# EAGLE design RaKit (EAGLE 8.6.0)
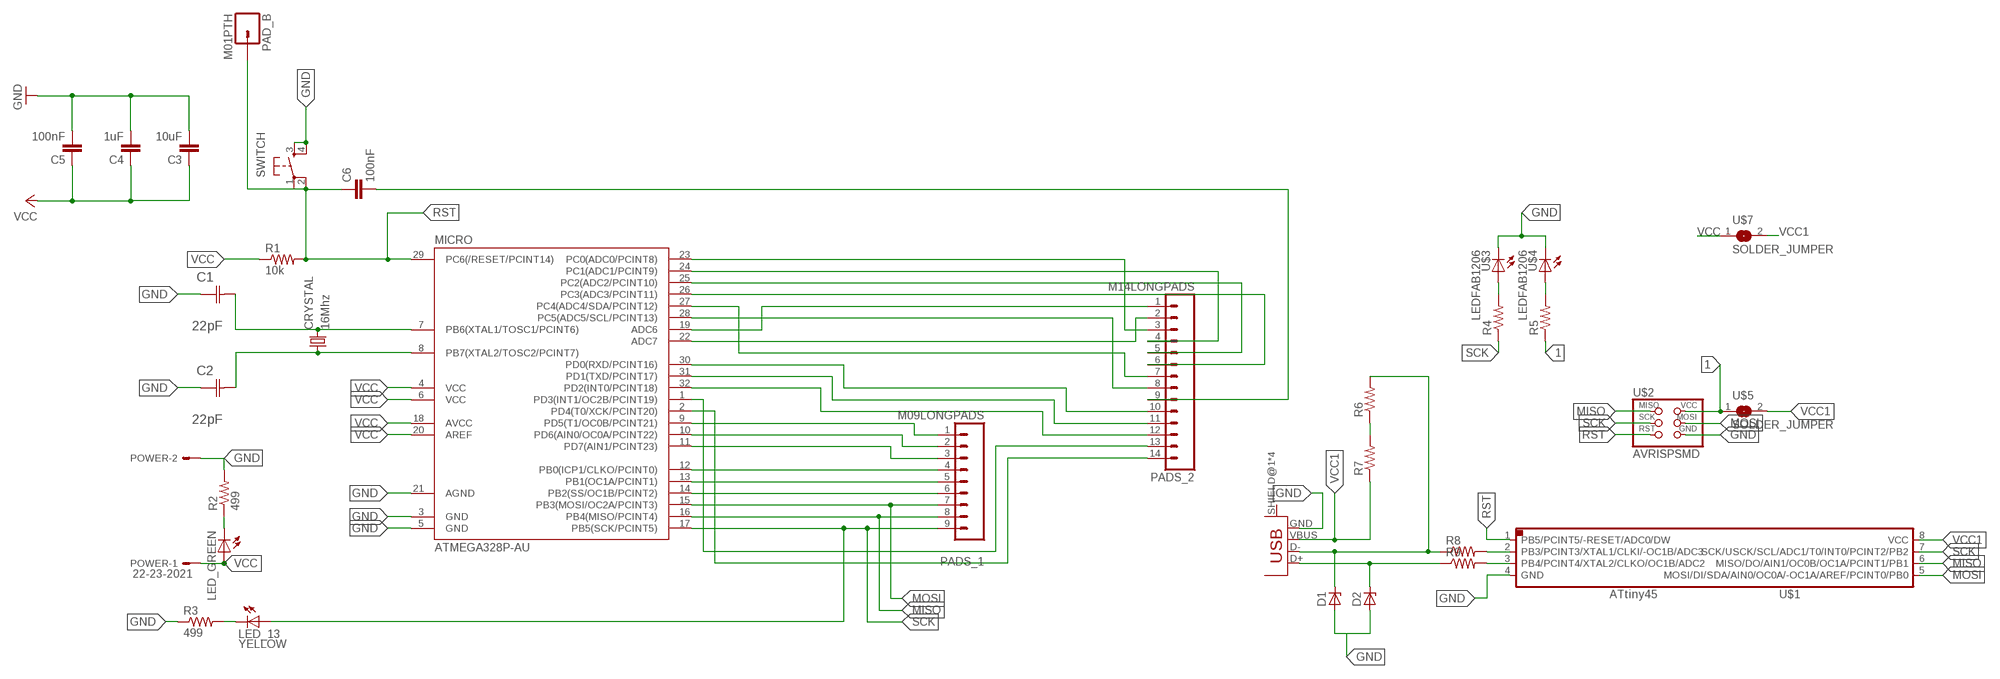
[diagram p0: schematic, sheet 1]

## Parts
C1  22pF  0612ZC225MAT2A  [CAPC3216X178N]
C2  22pF  0612ZC225MAT2A  [CAPC3216X178N]
C3  10uF  CAP1206  [1206]
C4  1uF  CAP1206  [1206]
C5  100nF  CAP1206  [1206]
C6  100nF  CAP1206  [1206]
CRYSTAL  16Mhz  CSM-7X-DU  [CSM-7X-DU]
D1  ZENER_DIODESOD123  [SOD123]
D2  ZENER_DIODESOD123  [SOD123]
LED_13  YELLOW  LED1206  [1206]
LED_GREEN  LED1206  [1206]
MICRO  ATMEGA328P-AU  ATMEGA48/88/168-AU  [TQFP32-08]
PAD_B  M01PTH  [1X01]
PADS_1  M09LONGPADS  [1X09_LONGPADS]
PADS_2  M14LONGPADS  [1X14-LONGPADS]
POWER  22-23-2021  [22-23-2021]
R1  10k  RESISTOR1206  [1206]
R2  499  RESISTOR1206  [1206]
R3  499  RESISTOR1206  [1206]
R4  RES-US1206FAB  [R1206FAB]
R5  RES-US1206FAB  [R1206FAB]
R6  RES-US1206FAB  [R1206FAB]
R7  RES-US1206FAB  [R1206FAB]
R8  RES-US1206FAB  [R1206FAB]
R9  RES-US1206FAB  [R1206FAB]
SWITCH  6MM_SWITCH6MM_SWITCH  [6MM_SWITCH]
U$1  ATTINY45SI  [SOIC8]
U$2  AVRISPSMD  [2X03SMD]
U$3  LEDFAB1206  [LED1206FAB]
U$4  LEDFAB1206  [LED1206FAB]
U$5  SOLDER_JUMPER  [SJFAB]
U$6  USB_MINIB  [USB_MINIB]
U$7  SOLDER_JUMPER  [SJFAB]

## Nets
1: R5.1 U$2.2(VCC) U$5.1
GND: C1.1(C1) C2.1(C1) C3.2 C4.2 C5.2 D1.ANODE D2.ANODE MICRO.3(GND) MICRO.5(GND) MICRO.21(AGND) POWER.2 R2.2 R3.1 SWITCH.3(S) SWITCH.4(S1) U$1.4(GND) U$2.6(GND) U$3.2(C) U$4.2(C) U$6.GND
MISO: MICRO.16(PB4(MISO/PCINT4)) PADS_1.8 U$1.6(MISO/DO/AIN1/OC0B/OC1A/PCINT1/PB1) U$2.1(MISO)
MOSI: MICRO.15(PB3(MOSI/OC2A/PCINT3)) PADS_1.7 U$1.5(MOSI/DI/SDA/AIN0/OC0A/-OC1A/AREF/PCINT0/PB0) U$2.4(MOSI)
N$1: MICRO.9(PD5(T1/OC0B/PCINT21)) PADS_1.1
N$2: C1.2(C2) CRYSTAL.2 MICRO.7(PB6(XTAL1/TOSC1/PCINT6))
N$3: C6.2 PADS_2.9
N$4: MICRO.10(PD6(AIN0/OC0A/PCINT22)) PADS_1.2
N$5: MICRO.11(PD7(AIN1/PCINT23)) PADS_1.3
N$6: MICRO.12(PB0(ICP1/CLKO/PCINT0)) PADS_1.4
N$7: MICRO.13(PB1(OC1A/PCINT1)) PADS_1.5
N$8: MICRO.14(PB2(SS/OC1B/PCINT2)) PADS_1.6
N$9: C2.2(C2) CRYSTAL.1 MICRO.8(PB7(XTAL2/TOSC2/PCINT7))
N$13: MICRO.19(ADC6) PADS_2.1
N$14: MICRO.22(ADC7) PADS_2.2
N$15: MICRO.23(PC0(ADC0/PCINT8)) PADS_2.3
N$16: MICRO.24(PC1(ADC1/PCINT9)) PADS_2.4
N$17: MICRO.25(PC2(ADC2/PCINT10)) PADS_2.5
N$18: MICRO.26(PC3(ADC3/PCINT11)) PADS_2.6
N$19: MICRO.27(PC4(ADC4/SDA/PCINT12)) PADS_2.7
N$20: MICRO.30(PD0(RXD/PCINT16)) PADS_2.10
N$21: MICRO.31(PD1(TXD/PCINT17)) PADS_2.11
N$22: MICRO.32(PD2(INT0/PCINT18)) PADS_2.12
N$23: MICRO.1(PD3(INT1/OC2B/PCINT19)) PADS_2.13
N$24: MICRO.2(PD4(T0/XCK/PCINT20)) PADS_2.14
N$25: MICRO.28(PC5(ADC5/SCL/PCINT13)) PADS_2.8
N$26: LED_GREEN.2(C) R2.1
N$27: LED_13.2(C) R3.2
N$29: D1.CATHODE R6.2 R8.1 U$6.D-
N$30: R8.2 U$1.2(PB3/PCINT3/XTAL1/CLKI/-OC1B/ADC3)
N$31: D2.CATHODE R9.1 U$6.D+
N$32: R9.2 U$1.3(PB4/PCINT4/XTAL2/CLKO/OC1B/ADC2)
N$33: R4.2 U$3.1(A)
N$34: R5.2 U$4.1(A)
N$37: R6.1 R7.2
RST: C6.1 MICRO.29(PC6(/RESET/PCINT14)) PAD_B.1 R1.2 SWITCH.1(P) SWITCH.2(P1) U$1.1(PB5/PCINT5/-RESET/ADC0/DW) U$2.5(RST)
SCK: LED_13.1(A) MICRO.17(PB5(SCK/PCINT5)) PADS_1.9 R4.1 U$1.7(SCK/USCK/SCL/ADC1/T0/INT0/PCINT2/PB2) U$2.3(SCK)
VCC: C3.1 C4.1 C5.1 LED_GREEN.1(A) MICRO.4(VCC) MICRO.6(VCC) MICRO.18(AVCC) MICRO.20(AREF) POWER.1 R1.1 U$7.1
VCC1: R7.1 U$1.8(VCC) U$5.2 U$6.VBUS U$7.2
Unconnected: U$6.SHIELD@1(SHIELD) U$6.SHIELD@2(SHIELD) U$6.SHIELD@3(SHIELD) U$6.SHIELD@4(SHIELD)

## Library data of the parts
C1 C2 = AVX_By_element14_Batch_1:0612ZC225MAT2A: Capacitor 1206; MPN: 0612ZC225MAT2A; OC_FARNELL: unknown; OC_NEWARK: 12N3209; SUPPLIER: AVX; TOLERANCE: ±20%; VALUE: 2.2µF; VOLTAGERATING: 10V
C3 = 01_SparkFun:CAP: Capacitor; MF: PANASONIC ELECTRONIC COMPONENTS; MPN: ECEA1HN100U; OC_FARNELL: 9696636
C4-C6 = 01_SparkFun:CAP: Capacitor; OC_FARNELL: unknown
CRYSTAL = 01_FAB_Hello:CSM-7X-DU: SMD CRYSTAL; OC_FARNELL: unknown; OC_NEWARK: unknown
D1 D2 = fab:ZENER_DIODE: zener diode; OC_FARNELL: unknown
LED_13 LED_GREEN = 01_FAB_Hello:LED; OC_FARNELL: unknown
MICRO = atmega8:ATMEGA48/88/168; OC_FARNELL: unknown
PAD_B = 01_SparkFun:M01: Header 1; OC_FARNELL: unknown
PADS_1 = 01_SparkFun:M09: Header 9 Standard 9-pin 0.1" header. Use with straight break away headers (SKU : PRT-00116), right angle break away headers (PRT-00553), swiss pins (PRT-00743), machine pins (PRT-00117), and female headers (PRT-00115).; OC_FARNELL: unknown
PADS_2 = 01_SparkFun:M14: Header 14 Standard 14-pin 0.1" header. Use with straight break away headers (SKU : PRT-00116), right angle break away headers (PRT-00553), swiss pins (PRT-00743), machine pins (PRT-00117), and female headers (PRT-00115).; OC_FARNELL: unknown
POWER = con-molex:22-23-2021: .100" (2.54mm) Center Header - 2 Pin; MF: MOLEX; MPN: 22-23-2021; OC_FARNELL: 1462926; OC_NEWARK: 25C3832
R1-R3 = 01_SparkFun:RESISTOR: Resistor; OC_FARNELL: unknown
R4-R9 = fab:RES-US: Resistor (US Symbol); OC_FARNELL: unknown
SWITCH = 01_FAB_Hello:6MM_SWITCH: OMRON SWITCH; OC_FARNELL: unknown
U$1 = fab:ATTINY45; OC_FARNELL: unknown
U$2 = fab:AVRISP; OC_FARNELL: unknown
U$3 U$4 = fab:LED: LED; OC_FARNELL: unknown
U$5 U$7 = fab:SOLDER_JUMPER; OC_FARNELL: unknown
U$6 = fab:USB_MINIB; OC_FARNELL: unknown

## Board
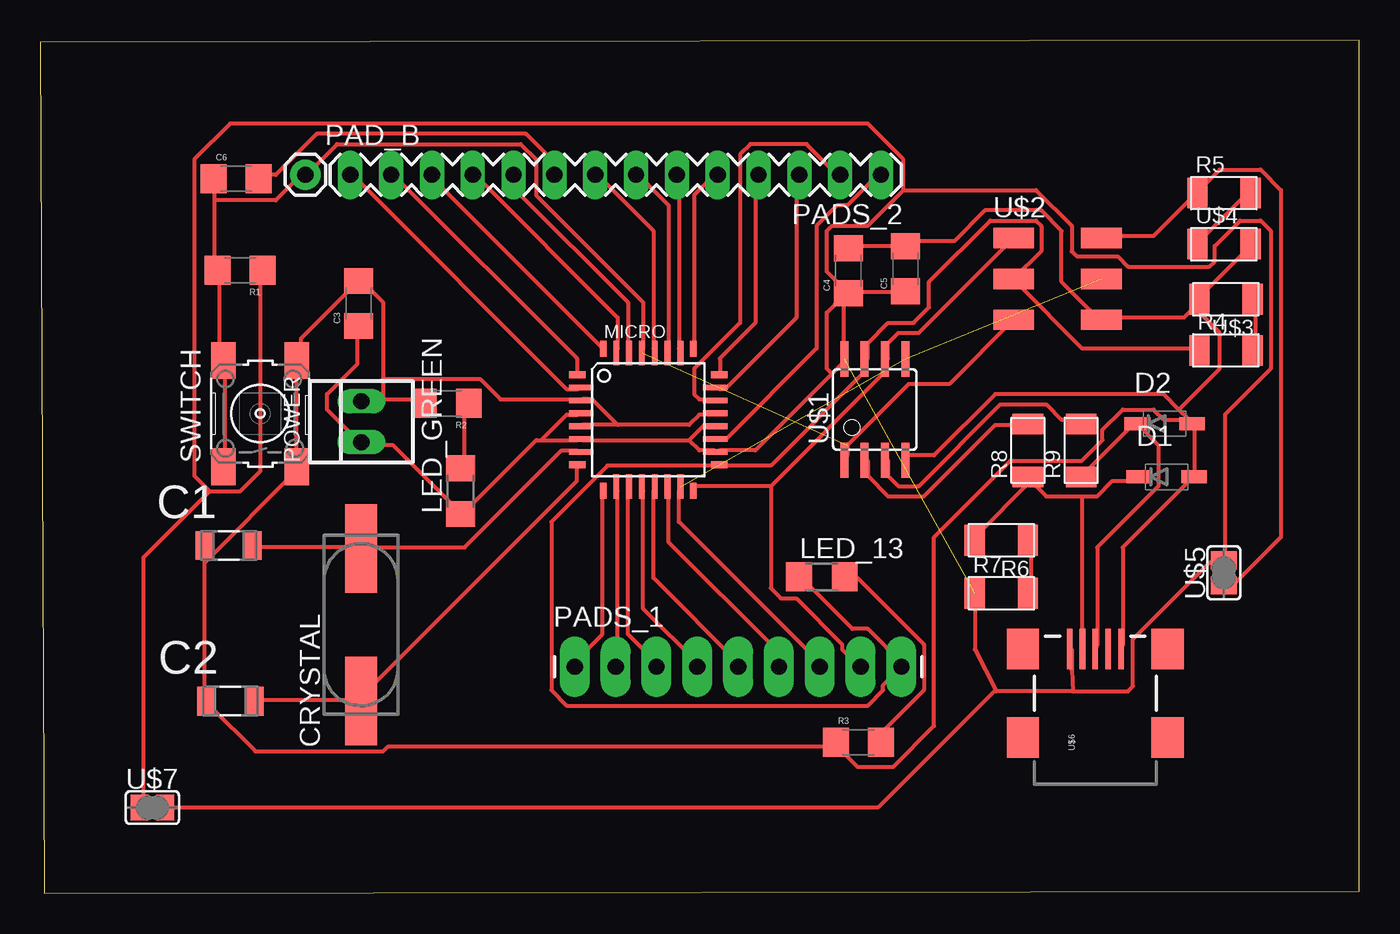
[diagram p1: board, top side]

Size 82.09 x 53.08 mm. Coordinates in mm from the lower left corner, seen from the top.
Outline: 0.25,0 82.09,0.13 82.09,53.08 0,52.95 0.25,0
Copper layers (1*16): Top 0.035mm / dielectric 1.5mm / Bottom 0.035mm
Design rules "default": minimum track width 10mil, minimum drill 24mil, track to track 8mil, track to pad 8mil, pad to pad 8mil, via to via 8mil, smd to smd 8mil, copper to edge 40mil, drill to drill 8mil, minimum pad ring 10mil, minimum via ring 8mil, stop-mask expansion 4mil, vias tented up to drill 0mil, thermal gap 10mil

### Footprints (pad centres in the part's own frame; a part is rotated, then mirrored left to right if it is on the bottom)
CAPC3216X178N = smd 1.118 x 1.803: 1 -1.499,0; 2 1.499,0
1206 = smd 1.6 x 1.8: 1 -1.4,0; 2 1.4,0
CSM-7X-DU = smd 5.5 x 2: 1 -4.75,0; 2 4.75,0
SOD123 = smd 1.6 x 0.8: ANODE 1.7,0; CATHODE -1.7,0
1206' = smd 1.6 x 1.803: 1 -1.422,0; 2 1.422,0
TQFP32-08 = smd 1.016 x 0.406: 1 -4.42,2.8; 8 -4.42,-2.8; 17 4.42,-2.8; 24 4.42,2.8 | smd 1.524 x 0.356: 2 -4.166,2; 3 -4.166,1.2; 4 -4.166,0.4; 5 -4.166,-0.4; 6 -4.166,-1.2; 7 -4.166,-2; 18 4.166,-2; 19 4.166,-1.2; 20 4.166,-0.4; 21 4.166,0.4; 22 4.166,1.2; 23 4.166,2 | smd 0.406 x 1.016: 9 -2.8,-4.42; 16 2.8,-4.42; 25 2.8,4.42; 32 -2.8,4.42 | smd 0.356 x 1.524: 10 -2,-4.166; 11 -1.2,-4.166; 12 -0.4,-4.166; 13 0.4,-4.166; 14 1.2,-4.166; 15 2,-4.166; 26 2,4.166; 27 1.2,4.166; 28 0.4,4.166; 29 -0.4,4.166; 30 -1.2,4.166; 31 -2,4.166
1X01 = drill 1.016 pad 1.88: 1 0,0
1X09_LONGPADS = drill 1.016 pad 1.88 long: 1 0,0; 2 2.54,0; 3 5.08,0; 4 7.62,0; 5 10.16,0; 6 12.7,0; 7 15.24,0; 8 17.78,0; 9 20.32,0
1X14-LONGPADS = drill 1.016 long: 1 0,0; 2 2.54,0; 3 5.08,0; 4 7.62,0; 5 10.16,0; 6 12.7,0; 7 15.24,0; 8 17.78,0; 9 20.32,0; 10 22.86,0; 11 25.4,0; 12 27.94,0; 13 30.48,0; 14 33.02,0
22-23-2021 = drill 1 long: 1 -1.27,0; 2 1.27,0
R1206FAB = smd 1.27 x 1.905: 1 -1.651,0; 2 1.651,0
6MM_SWITCH = smd 2.286 x 1.524: 1 -3.302,2.286; 2 3.302,2.286; 3 -3.302,-2.286; 4 3.302,-2.286
SOIC8 = smd 0.5 x 2.2: 1 -1.905,-3.154; 2 -0.645,-3.154; 3 0.625,-3.154; 4 1.895,-3.154; 5 1.905,3.154; 6 0.635,3.154; 7 -0.635,3.154; 8 -1.905,3.154
2X03SMD = smd 2.54 x 1.27: 1 -2.54,2.54; 2 2.92,2.54; 3 -2.54,0; 4 2.92,0; 5 -2.54,-2.54; 6 2.92,-2.54
LED1206FAB = smd 1.27 x 1.905: 1 -1.651,0; 2 1.651,0
SJFAB = smd 1.118 x 1.6: 1 -0.787,0; 2 0.787,0
USB_MINIB = smd 2.5 x 0.35: D+ 3.77,0; D- 3.77,0.8; GND 3.77,-1.6; ID 3.77,-0.8; VBUS 3.77,1.6 | smd 2.5 x 2: SHIELD@1 -1.73,-4.5; SHIELD@2 -1.73,4.5; SHIELD@3 3.77,4.5; SHIELD@4 3.77,-4.5

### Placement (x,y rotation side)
C1  11.73,21.64 0 top
C2  11.84,11.96 0 top
C3  19.81,36.7 90 top
C4  50.29,38.73 90 top
C5  53.85,38.86 90 top
C6  12.19,44.45 0 top
CRYSTAL  19.96,16.71 90 top
D1  70.1,25.91 0 top
D2  69.98,29.21 0 top
LED_13  YELLOW  [1206']  48.64,19.69 0 top
LED_GREEN  [1206']  26.16,25.02 90 top
MICRO  37.85,29.46 0 top
PAD_B  16.51,44.7 0 top
PADS_1  33.27,14.1 0 top
PADS_2  52.32,44.7 180 top
POWER  19.99,29.34 90 top
R1  12.45,38.76 180 top
R2  25.27,30.48 180 top
R3  50.93,9.4 0 top
R4  73.79,33.78 0 top
R5  73.66,43.56 0 top
R6  59.82,21.97 180 top
R7  59.82,18.67 0 top
R8  61.47,27.56 90 top
R9  64.77,27.56 90 top
SWITCH  13.69,29.84 90 top
U$1  51.94,30.1 0 top
U$2  63.12,38.23 0 top
U$3  73.79,36.96 180 top
U$4  73.66,40.39 0 top
U$5  73.66,19.94 90 top
U$6  65.66,11.43 90 top
U$7  6.99,5.33 0 top

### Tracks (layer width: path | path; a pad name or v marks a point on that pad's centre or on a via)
1
  Top 0.254: U$5.1 73.72,19.3 74.36,19.3 77.22,22.16 77.22,43.75 75.95,45.02 73.41,45.02 72.14,43.75 R5.1 71.82,43.43 69.28,40.89 66.1,40.89 U$2.2
GND
  Top 0.254: C4.2 50.55,40.26 53.72,40.26 C5.2 54.04,40.58 56.9,40.58 58.8,42.48 62.29,42.48 63.56,41.21 63.56,38.04 65.79,35.81 U$2.6 66.1,35.81 71.18,35.81 71.82,36.45 | U$3.2 72.14,37.08 75.31,40.26 U$4.2 | 71.82,36.45 72.14,36.77 U$3.2 | 71.5,29.46 70.87,30.1 | 70.87,30.1 69.91,31.05 59.44,31.05 55.63,27.24 54.04,27.24 U$1.4 | U$6.GND 67.37,15.49 67.37,21.53 71.5,25.65 D1.ANODE 71.82,25.97 71.82,29.15 D2.ANODE 71.5,29.46 | 71.82,36.45 73.41,34.86 73.41,32.64 70.87,30.1 | 71.82,36.45 U$3.2 | 35.94,29.15 40.39,29.15 41.02,29.78 41.97,29.78 MICRO.21 | 35.94,29.15 33.72,29.15 MICRO.5 | 35.94,29.15 34.35,30.73 33.72,30.73 MICRO.3 33.4,30.73 28.64,30.73 27.37,32 21.34,32 | 21.34,30.73 20.07,30.73 POWER.2 21.34,30.73 | 21.34,30.73 23.56,30.73 R2.2 | 21.34,32 21.34,36.77 20.07,38.04 C3.2 19.75,38.04 16.26,34.54 16.26,33.27 SWITCH.4 15.94,32.96 15.94,26.61 SWITCH.3 15.94,26.29 10.22,20.57 | 21.34,32 21.34,30.73 | 10.22,20.57 10.22,12 C2.1 10.54,11.68 13.4,8.83 21.34,8.83 21.65,9.14 49.28,9.14 R3.1 49.59,9.14 50.86,7.87 53.09,7.87 55.63,10.41 55.63,22.16 60.39,26.92 64.83,26.92 66.1,28.19 66.1,28.83 67.37,30.1 69.28,30.1 69.91,29.46 71.5,29.46 | 10.22,20.57 10.22,21.53 C1.1
MISO
  Top 0.254: 45.47,25.34 40.7,25.34 MICRO.16 | 45.47,25.34 52.45,32.32 52.45,32.96 U$1.6 52.77,33.27 52.77,34.23 53.4,34.86 54.67,34.86 U$2.1 | 45.47,25.34 45.47,18.99 46.1,18.35 47.05,18.35 49.91,15.49 49.91,15.18 50.86,14.22 PADS_1.8
MOSI  (2 unrouted)
  Top 0.254: MICRO.15 39.75,25.02 39.75,23.11 48.64,14.22 PADS_1.7
N$1
  Top 0.254: MICRO.9 34.99,25.02 34.99,16.13 33.08,14.22 PADS_1.1
N$2
  Top 0.254: MICRO.7 33.4,27.56 32.45,27.56 26.42,21.53 20.07,21.53 CRYSTAL.2 19.75,21.53 13.4,21.53 C1.2
N$3
  Top 0.254: C6.2 13.72,44.7 14.67,44.7 17.21,47.24 30.23,47.24 31.81,45.66 31.81,44.7 PADS_2.9
N$4
  Top 0.254: MICRO.10 35.94,25.02 35.94,14.22 PADS_1.2
N$5
  Top 0.254: MICRO.11 36.58,25.02 36.58,16.13 38.48,14.22 PADS_1.3
N$6
  Top 0.254: MICRO.12 37.53,25.02 37.53,17.72 41.02,14.22 PADS_1.4
N$7
  Top 0.254: MICRO.13 38.16,25.02 38.16,19.62 43.56,14.22 PADS_1.5
N$8
  Top 0.254: MICRO.14 39.12,25.02 39.12,21.84 45.78,15.18 45.78,14.22 PADS_1.6
N$9
  Top 0.254: 19.75,12 33.4,25.65 33.4,26.61 MICRO.8 | 19.75,12 13.4,12 C2.2 | 19.75,12 CRYSTAL.1
N$13
  Top 0.254: MICRO.19 42.29,28.19 42.61,28.19 48.32,33.91 48.32,41.53 49.59,42.8 50.23,42.8 52.13,44.7 PADS_2.1
N$14
  Top 0.254: MICRO.22 41.97,30.73 41.02,30.73 40.7,31.05 40.7,32.64 43.56,35.5 43.56,45.97 44.2,46.61 47.69,46.61 49.59,44.7 PADS_2.2
N$15
  Top 0.254: MICRO.23 42.29,31.37 42.61,31.37 47.05,35.81 47.05,44.7 PADS_2.3
N$16
  Top 0.254: MICRO.24 42.29,32.32 42.29,33.27 44.51,35.5 44.51,44.7 PADS_2.4
N$17
  Top 0.254: MICRO.25 40.7,33.91 40.7,43.43 41.97,44.7 PADS_2.5
N$18
  Top 0.254: MICRO.26 39.75,33.91 39.75,44.7 PADS_2.6
N$19
  Top 0.254: MICRO.27 39.12,33.91 39.12,42.8 37.21,44.7 PADS_2.7
N$20
  Top 0.254: MICRO.30 36.58,33.91 36.58,36.77 29.59,43.75 29.59,44.7 PADS_2.10
N$21
  Top 0.254: MICRO.31 35.94,33.91 35.94,35.81 27.05,44.7 PADS_2.11
N$22
  Top 0.254: MICRO.32 34.99,33.91 24.19,44.7 PADS_2.12
N$23
  Top 0.254: MICRO.1 33.4,32.32 33.4,33.27 21.97,44.7 PADS_2.13
N$24
  Top 0.254: MICRO.2 33.4,31.37 32.77,31.37 19.43,44.7 PADS_2.14
N$25
  Top 0.254: MICRO.28 38.16,33.91 38.16,41.21 34.67,44.7 PADS_2.8
N$26
  Top 0.254: R2.1 26.42,30.42 26.42,26.61 LED_GREEN.2
N$27
  Top 0.254: R3.2 52.45,9.46 52.45,10.1 54.99,12.64 54.99,15.49 50.86,19.62 50.23,19.62 LED_13.2
N$29
  Top 0.254: 64.83,24.7 62.61,24.7 61.66,25.65 | 64.83,24.7 65.79,24.7 66.74,25.65 68.33,25.65 D1.CATHODE | 61.66,25.65 58.17,22.16 R6.2 | 61.66,25.65 R8.1 | 64.83,24.7 64.83,15.49 U$6.D-
N$30
  Top 0.254: R8.2 61.34,29.15 59.44,29.15 54.99,24.7 52.77,24.7 51.5,25.97 51.5,26.92 U$1.2
N$31
  Top 0.254: R9.1 68.01,29.15 D2.CATHODE 68.33,29.15 69.6,27.88 69.6,25.34 65.79,21.53 65.79,15.49 U$6.D+
N$32
  Top 0.254: R9.2 64.52,29.46 63.56,29.46 62.61,30.42 59.75,30.42 54.67,25.34 53.4,25.34 52.77,25.97 52.77,26.92 U$1.3
N$33
  Top 0.254: R4.2 75.63,33.91 75.63,36.77 U$3.1
N$34
  Top 0.254: U$4.1 72.14,40.58 75.31,43.75 R5.2
N$37
  Top 0.254: R7.2 61.66,18.67 61.66,21.84 R6.1
RST  (1 unrouted)
  Top 0.254: U$2.5 56.58,31.69 54.04,31.69 50.23,27.88 50.23,27.24 U$1.1 | 10.86,43.12 10.86,38.99 R1.2 11.18,38.67 11.18,33.27 SWITCH.2 11.49,32.96 11.49,26.61 SWITCH.1 | 10.86,43.12 10.86,44.39 C6.1 | MICRO.29 37.53,33.91 37.53,36.77 30.86,43.43 30.86,45.66 29.91,46.61 18.48,46.61 16.57,44.7 PAD_B.1 16.26,44.7 14.67,43.12 10.86,43.12
SCK
  Top 0.254: R4.1 72.14,33.91 64.83,33.91 60.71,38.04 U$2.3 62.29,39.94 62.29,41.53 61.98,41.85 59.12,41.85 55.31,38.04 55.31,36.45 54.36,35.5 52.77,35.5 51.5,34.23 51.5,33.27 U$1.7 51.18,32.96 51.18,32.32 45.47,26.61 42.29,26.61 MICRO.17 41.97,26.61 35.31,26.61 31.81,23.11 31.81,12.64 32.77,11.68 51.5,11.68 52.45,12.64 52.45,12.95 PADS_1.9 53.72,14.22 51.5,16.45 50.55,16.45 47.37,19.62 LED_13.1
VCC
  Top 0.254: C3.1 19.75,35.18 19.75,32.96 17.84,31.05 17.84,30.1 19.75,28.19 POWER.1 20.07,27.88 21.97,27.88 26.1,23.75 LED_GREEN.1 26.42,23.75 30.86,28.19 31.18,28.19 | 31.18,28.19 33.4,28.19 MICRO.6 33.72,28.19 40.39,28.19 | 40.39,28.19 41.34,29.15 41.97,29.15 MICRO.20 | 31.18,28.19 32.77,29.78 33.4,29.78 MICRO.4 | 49.91,32.96 49.28,32.32 | 49.28,32.32 44.51,27.56 42.29,27.56 MICRO.18 41.97,27.56 41.02,27.56 40.39,28.19 | C4.1 50.55,37.4 53.72,37.4 C5.1 | 10.54,25.02 12.45,25.02 13.72,26.29 13.72,38.67 R1.1 | 10.54,25.02 9.59,25.97 9.59,45.66 11.81,47.88 51.5,47.88 53.72,45.66 53.72,43.75 | 53.72,43.75 51.5,41.53 49.28,41.53 48.96,41.21 48.96,38.67 50.23,37.4 C4.1 | 49.97,33.15 49.97,36.96 C4.1 | 73.72,20.89 73.72,29.78 76.58,32.64 76.58,41.21 75.95,41.85 74.68,41.85 73.09,40.26 73.09,39.31 72.77,38.99 67.69,38.99 67.06,39.62 64.52,39.62 64.2,39.94 64.2,41.53 61.98,43.75 53.72,43.75 | 10.54,25.02 6.41,20.89 6.41,5.33 U$7.1 | 49.28,32.32 48.96,32.64 48.96,36.13 49.91,37.08 50.23,37.08 C4.1
VCC1  (1 unrouted)
  Top 0.254: 64.26,12.57 67.69,12.57 68.01,12.89 68.01,15.81 72.77,20.57 73.41,20.57 U$5.2 | 64.26,12.57 64.2,13.91 64.2,15.18 U$6.VBUS | 59.46,12.65 58.17,15.18 R7.1 | 59.46,12.65 59.5,12.57 64.26,12.57 | U$7.2 52.13,5.33 59.44,12.64 59.46,12.65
